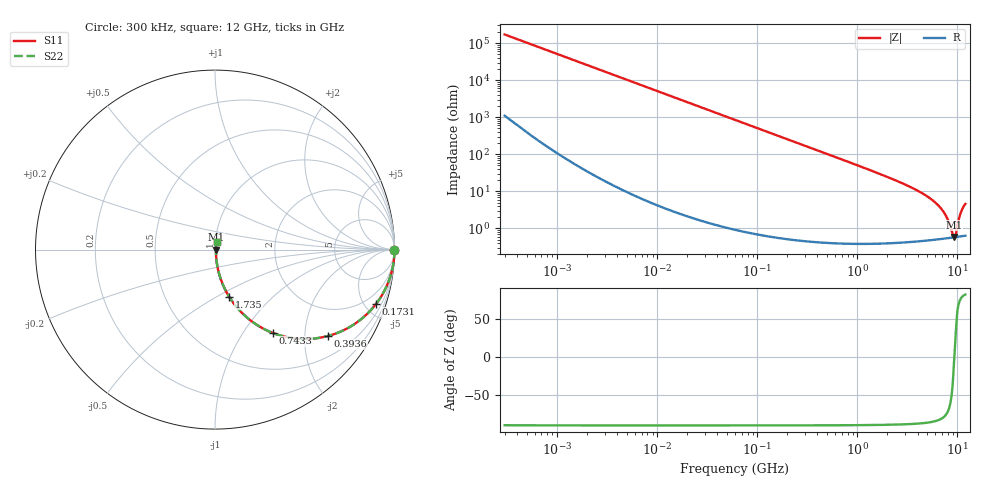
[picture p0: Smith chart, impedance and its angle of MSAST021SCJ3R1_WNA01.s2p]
! MSAST021SCJ3R1_WNA01  S-PARAMETER MODEL  ( General Type )
! Model Generated by TAIYO YUDEN Corporation (http://www.ty-top.com)
! Version 2.0
! TAIYO YUDEN Control No. 181101
! Copyright(c) 2015 TAIYO YUDEN CO.,LTD. All Rights Reserved.
! Product Description (link to TY-COMPAS)
! https://ds.yuden.co.jp/TYCOMPAS/or/detail?pn=MSAST021SCJ3R1BWNA01&u=M
! Products Name : Multilayer Ceramic Capacitors
! Characteristics :
!  Capacitance : 3.1 pF , Rated Voltage : 25V , TCC : CJ / C0J
!  Case Size : 0.25 x 0.125 / 0.0098 x 0.0049 [mm/inch] , Thickness : 0.125 / 0.0049 [mm/inch]
!  (Conditions: Temperature = 25 degC , DC Bias Current/Voltage = 0A / 0V)
! External Node Assignments :
!  1  o---| |---o  2
! GND o---------o GND
! Frequency Range : 0.3MHz  -  12000MHz  [ 401 STEP ]
# MHz S RI R 50
! Freq[MHz].  S11 Real  S11 Imag  S21 Real  S21 Imag  S12 Real  S12 Imag  S22 Real  S22 Imag
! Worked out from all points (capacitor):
!   401 points, 300 kHz to 12 GHz, reference 50 ohm
!   read as one part in series: C = 3.1 pF near 316.3 kHz
!   lowest |Z| = 588 mohm at 9.207 GHz (marker M1)
!   series resonance near 9.312 GHz, so ESL is about 94 pH
!   S11 on the Smith chart (normalised r, x): 300 kHz: open; 173.1 MHz: 1.01, -5.93; 393.6 MHz: 1.01, -2.60; 743.3 MHz: 1.01, -1.37; 1.735 GHz: 1.01, -0.57; 12 GHz: 1.01, +0.09
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0.3  1 -0.000584  4.11e-06 0.000584  4.11e-06 0.000584  1 -0.000584
1.769972  1 -0.00345  1.69e-05 0.00345  1.69e-05 0.00345  1 -0.00345
10.44266  0.9996 -0.0203  0.00043 0.0203  0.00043 0.0203  0.9996 -0.0203
60  0.9864 -0.1153  0.0136 0.1153  0.0136 0.1153  0.9864 -0.1153
173.124  0.8974 -0.3025  0.1026 0.3025  0.1026 0.3025  0.8974 -0.3025
353.9943  0.6766 -0.4663  0.3234 0.4663  0.3234 0.4663  0.6766 -0.4663
393.5654  0.6286 -0.4815  0.3714 0.4815  0.3714 0.4815  0.6286 -0.4815
743.2595  0.3212 -0.4641  0.6788 0.4641  0.6788 0.4641  0.3212 -0.4641
1135.593  0.1677 -0.3693  0.8323 0.3693  0.8323 0.3693  0.1677 -0.3693
1735.023  0.0785 -0.2622  0.9215 0.2622  0.9215 0.2622  0.0785 -0.2622
2088.533  0.0551 -0.2197  0.9449 0.2197  0.9449 0.2197  0.0551 -0.2197
3944.255  0.0156 -0.1046  0.9844 0.1046  0.9844 0.1046  0.0156 -0.1046
5868.704  0.00765 -0.052  0.9923 0.052  0.9923 0.052  0.00765 -0.052
6699.894  0.00647 -0.0365  0.9935 0.0365  0.9935 0.0365  0.00647 -0.0365
7448.838  0.00592 -0.0245  0.9941 0.0245  0.9941 0.0245  0.00592 -0.0245
8064.993  0.00571 -0.0156  0.9943 0.0156  0.9943 0.0156  0.00571 -0.0156
8966.534  0.00569 -0.00403  0.9943 0.00403  0.9943 0.00403  0.00569 -0.00403
9207.246  0.00573 -0.00113  0.9943 0.00113  0.9943 0.00113  0.00573 -0.00113
9708.23  0.00587 0.00485  0.9941 -0.00485  0.9941 -0.00485  0.00587 0.00485
10511.28  0.00644 0.0203  0.9936 -0.0203  0.9936 -0.0203  0.00644 0.0203
11083.22  0.00711 0.0309  0.9929 -0.0309  0.9929 -0.0309  0.00711 0.0309
12000  0.00838 0.0449  0.9916 -0.0449  0.9916 -0.0449  0.00838 0.0449
